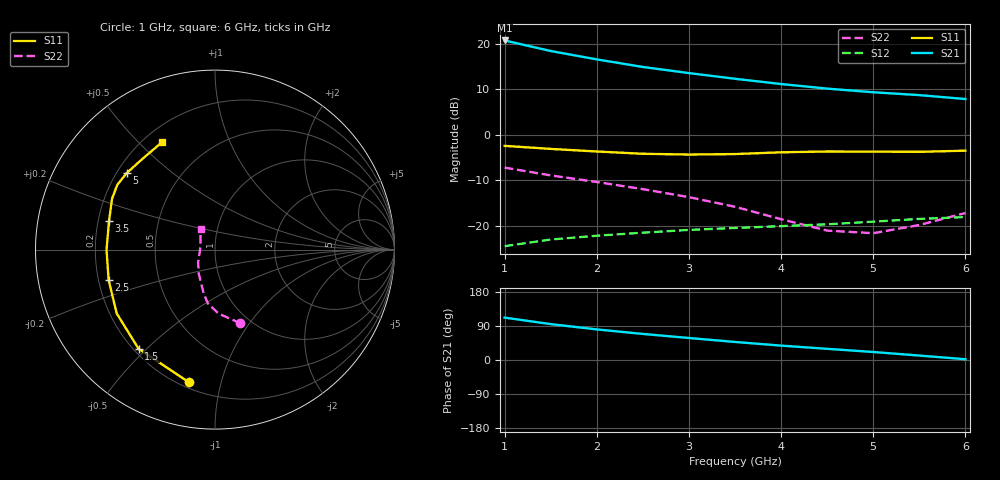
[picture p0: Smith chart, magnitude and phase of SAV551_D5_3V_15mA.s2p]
! Created Mon Oct 27 14:25:13 2008
# hz S ma R 50
! 2 Port Network Data from SP1.SP block
! freq  magS11  angS11  magS21  angS21  magS12  angS12  magS22  angS22
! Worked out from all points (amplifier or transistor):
!   11 points, 1 GHz to 6 GHz, reference 50 ohm
!   highest |S21| = 20.7 dB at 1 GHz (marker M1)
!   |S21| within 3 dB of that: start of sweep to 1.685 GHz
!   unconditionally stable (mu >= 1): 4.595 GHz to end of sweep
!   at 1.5 GHz: K = 0.44, MSG = 20.7 dB, |S12| = -23.0 dB
!   at 3.5 GHz: K = 0.89, MSG = 16.4 dB, |S12| = -20.5 dB
!   at 6 GHz: K = 1.08, MAG = 11.2 dB, |S12| = -18.1 dB
!   S11 on the Smith chart (normalised r, x): 1 GHz: 0.23, -0.80; 1.5 GHz: 0.22, -0.47; 2.5 GHz: 0.24, -0.13; 3.5 GHz: 0.24, +0.13; 5 GHz: 0.24, +0.35; 6 GHz: 0.27, +0.59
1e9  0.7532 -101.2  10.82 111.9  0.05962 39.2  0.4345 -71.0
1.5e9  0.6975 -127.6  8.286 94.7  0.07051 30.8  0.3569 -86.8
2e9  0.653 -147.0  6.704 80.7  0.07766 24.6  0.3021 -97.6
2.5e9  0.6164 -164.0  5.534 68.8  0.08386 20.0  0.2521 -104.5
3e9  0.6044 -179.9  4.743 58.1  0.08997 16.6  0.206 -111.7
3.5e9  0.612 164.7  4.107 47.6  0.09439 12.5  0.1615 -124.1
4e9  0.64 153.6  3.595 37.9  0.09901 9.0  0.1179 -143.0
4.5e9  0.6531 146.5  3.203 29.5  0.1037 7.1  0.08834 -166.7
5e9  0.6511 139.2  2.921 21.1  0.1108 4.0  0.08278 167.7
5.5e9  0.6474 128.4  2.716 11.7  0.1189 -0.2  0.1018 143.2
6e9  0.6668 116.5  2.462 2.0  0.1244 -5.1  0.1378 125.3
